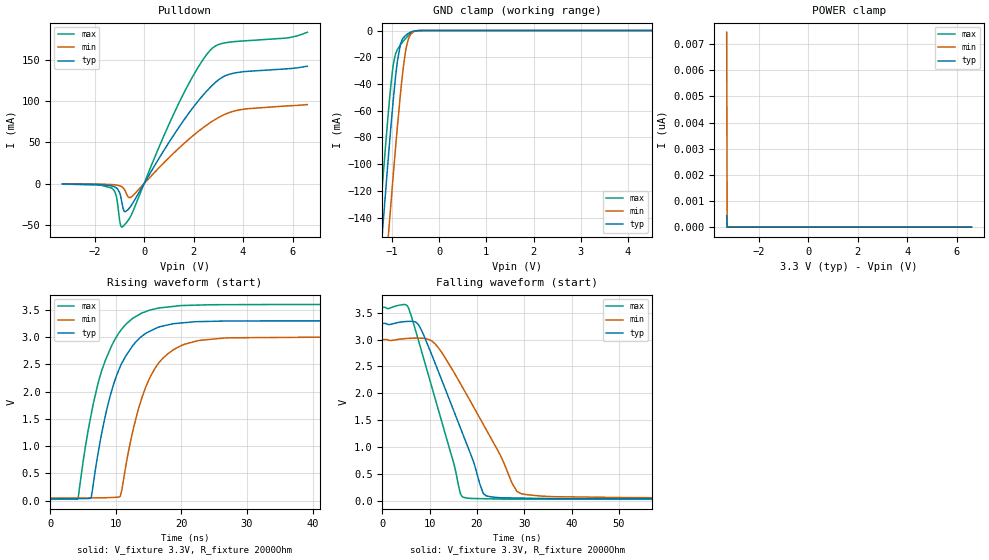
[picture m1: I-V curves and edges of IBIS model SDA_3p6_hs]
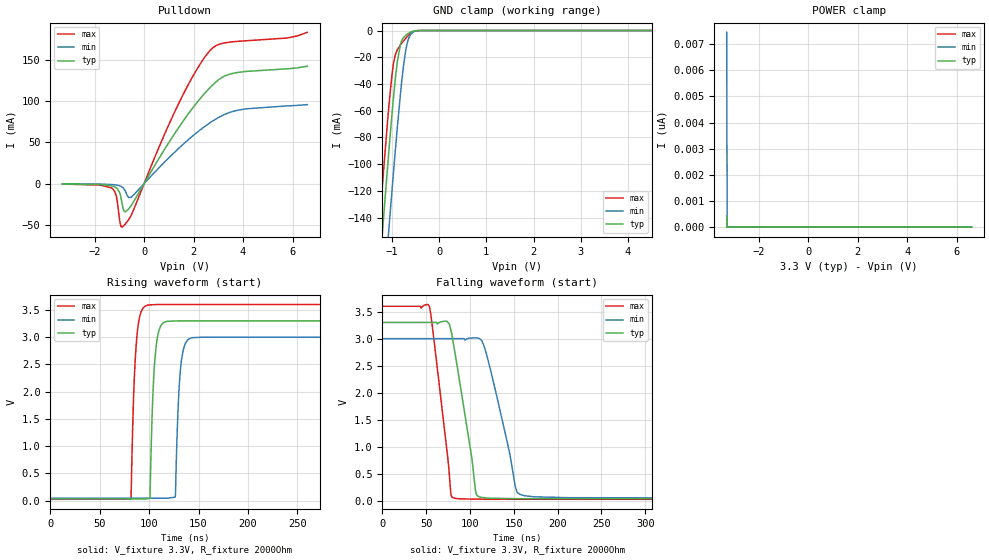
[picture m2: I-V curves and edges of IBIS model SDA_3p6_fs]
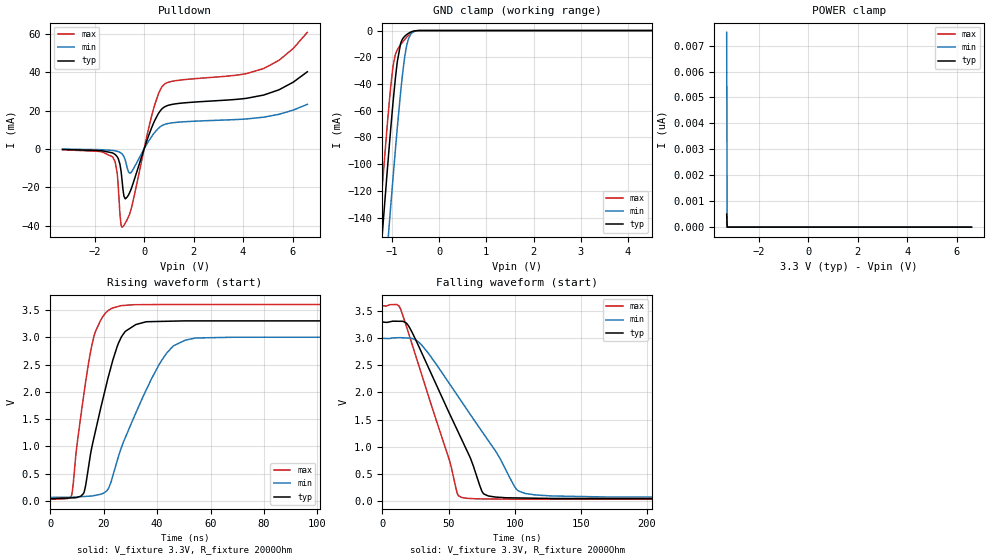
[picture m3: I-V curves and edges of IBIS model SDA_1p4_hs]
|Texas Instruments Incorporated
| Digital Temperature Sensor with Two-Wire Interface and Alert
| Marketing part#   Digital Voltage Range
| TMP75C   1.4V - 3.6V
[IBIS Ver]   4.1
[File name]   tmp75c.ibs
[File Rev]   1.0
[Date]   03/07/2014
[Source]
| Texas Instruments Incorporated.
| 12500 TI Blvd
| Dallas, TX -75243
[Notes]   Revision History:
| Rev 1.1: 09/17/2018
| - SDA_3p6_hs and SDA_3p6_fs models updated.
| Rev 1.0: 03/07/2014
| - Initial version of the model
| - Model generated from simulations in TISPICE
| - C_comp although listed in numerical order of value are
|   obtained from varying PVT conditions. For PVT conditions for
|   each specific value refer the buffer description under
|   respective [Model]. IBIS model user is responsible for using
|   appropriate C_comp to simulate for Signal Integrity.
| - Warnings regarding combined Non-monotonicity of various models have been
|   reviewd and considered minor and can be ignored.
| - Model names with a trailing _1p4 contains the model for
|   1.4V operation.Model names with a trailing _3p6 contains the model
|   for 3.6V operation.
[Disclaimer]
| This model is designed as an aid for customers of Texas Instruments.
| TI and its licensors and suppliers make no warranties, either expressed
| or implied, with respect to this  model, including the warranties of
| merchantability or fitness for a particular purpose. The model is
| provided solely on an "as is" basis. The entire risk as to its quality
| and performance is with the customer.
[Copyright]
 (C) Copyright 2014 Texas Instruments Incorporated.All rights reserved.
|   Device
[Component]   TMP75C
[Manufacturer]   TI
[Package]
| variable   typ   min   max
R_pkg   0.083   0.076   0.088
L_pkg   1.774nH   1.670nH   1.869nH
C_pkg   0.393pF   0.385pF   0.402pF
[Pin]  signal_name   model_name   R_pin   L_pin   C_pin
1   SDA   SDA   0.08836   1.8688nH   0.38537pF
2   SCL   SCL   0.0798   1.72452nH   0.40219pF
3   ALERT   ALERT   0.07626   1.67019nH   0.40077pF
4   GND   GND   0.08804   1.86388nH   0.38801pF
5   A2   A1   0.08833   1.8612nH   0.38619pF
6   A1   A1   0.07742   1.67952nH   0.40007pF
7   A0   A0   0.07743   1.67952nH   0.40011pF
8   V+   POWER   0.08723   1.84409nH   0.38521pF
|   Model Selectors
[Model Selector]  SDA
SDA_3p6_fs   SDA buffer at 3.6V with fast mode.
SDA_3p6_hs   SDA buffer at 3.6V with high speed mode.
SDA_1p4_fs   SDA buffer at 1.4V with fast mode.
SDA_1p4_hs   SDA buffer at 1.4V with high speed mode.
[Model Selector]  SCL
SCL_3p6   SCL buffer at 3.6V.
SCL_1p4   SCL buffer at 1.4V.
[Model Selector]  ALERT
ALERT_3p6   SCL buffer at 3.6V.
ALERT_1p4   SCL buffer at 1.4V.
[Model Selector]  A1
A1_3p6   A1/A2 buffer at 3.6V.
A1_1p4   A1/A2 buffer at 1.4V.
[Model Selector]  A0
A0_3p6   A0 buffer at 3.6V.
A0_1p4   A0 buffer at 1.4V.
| Models and submodels in the file (12): SDA_3p6_hs (I/O_open_drain), SDA_3p6_fs (I/O_open_drain), SDA_1p4_hs (I/O_open_drain), SDA_1p4_fs (I/O_open_drain), SCL_3p6 (Input), SCL_1p4 (Input), ALERT_3p6 (Open_drain), ALERT_1p4 (Open_drain), A1_3p6 (Input), A1_1p4 (Input), A0_3p6 (Input), A0_1p4 (Input)
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|   Model
[Model]   SDA_3p6_hs
Model_type   I/O_open_drain
Polarity   Non-Inverting
Enable   Active-Low
Vinl = 0.5
Vinh = 1.4
Vmeas = 1.65
Vref = 3.3
Cref = 1pF
Rref = 2000
|   typ   min   max
C_comp   0.767pF   0.704pF   0.863pF
[Voltage Range]   3.3   3   3.6
[Temperature Range]   25   125   -40
[Pullup Reference]   3.3   3   3.6
[Pulldown Reference]   0   0   0
[Power Clamp Reference]   3.3   3   3.6
[GND Clamp Reference]   0   0   0
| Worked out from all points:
|   slope of the pulldown table from 0 to 0.495 V, typ, clamps not added: 19.6 ohm
|   GND clamp passes 1 mA (typ) near -0.59 V on its own axis
|   falling waveform, V_fixture 3.3V, R_fixture 2000Ohm: 20-80 % time 8.64ns typ, 11ns min, 7ns max; typ from 3.3 V to 0.031 V
|   rising waveform, V_fixture 3.3V, R_fixture 2000Ohm: 20-80 % time 4.43ns typ, 4.36ns min, 4.49ns max; typ from 0.032 V to 3.3 V
[Pulldown]
|   Voltage   I(typ)   I(min)   I(max)
-3.3V     -437.4uA   -247.2uA   -600.7uA
-1.3V     -2.881mA   -1.227mA   -5.604mA
-1.122V   -5.223mA   -1.809mA   -15.61mA
-973.5mV  -12.58mA   -2.879mA   -47.55mA
-894.3mV  -23.64mA   -4.05mA    -52.74mA
-765.6mV  -34.14mA   -8.745mA   -49.02mA
-518.1mV  -26.42mA   -16.28mA   -38.03mA
1.304V    63.54mA    39.9mA     90.99mA
2.095V    96.47mA    60.83mA    136.3mA
2.68V     116.6mA    73.83mA    161.5mA
3.62V     133.5mA    87.51mA    171.6mA
6.6V      141.9mA    95.47mA    182.9mA
[GND Clamp]
|   Voltage   I(typ)   I(min)   I(max)
-3.3V     -1.174A    -1.231A    -1.141A
-1.29V    -193.5mA   -253.4mA   -157.8mA
-1.251V   -175.1mA   -235mA     -139.4mA
-1.191V   -147.7mA   -207.5mA   -112.3mA
-1.063V   -90.37mA   -149.1mA   -57.03mA
-963.6mV  -49.9mA    -105.8mA   -24.49mA
-884.4mV  -23.47mA   -73.04mA   -14.42mA
-815.1mV  -9.936mA   -46.83mA   -10.7mA
-755.7mV  -5.477mA   -27.58mA   -7.962mA
-696.3mV  -3.35mA    -13.32mA   -5.458mA
-587.4mV  -990.5uA   -2.271mA   -1.777mA
6.6V      0A         0A         0A
[POWER Clamp]
|   Voltage   I(typ)   I(min)   I(max)
-3.3V     435.8pA    7.448nA    127.3pA
-3.28V    0A         0A         0A
-3.27V    0A         0A         0A
6.6V      0A         0A         0A
[Ramp]
R_load = 2000
|   typ   min   max
dV/dt_r   1.96106/4.42647e-09   1.77266/4.35501e-09   2.14571/4.48923e-09
dV/dt_f   1.96115/8.64404e-09   1.77274/1.09923e-08   2.14582/6.99294e-09
[Falling Waveform]
V_fixture = 3.3V
V_fixture_min = 3V
V_fixture_max = 3.6V
R_fixture = 2000Ohm
C_fixture = 0F
|   Time   V(typ)   V(min)   V(max)
0s        3.3V       3V         3.6V
5.492ns   3.338V     3.022V     3.594V
8.291ns   3.169V     3.025V     2.781V
11.4ns    2.502V     2.894V     1.825V
16.49ns   1.357V     2.18V      127.8mV
18.36ns   933.5mV    1.891V     43.02mV
21.91ns   89.91mV    1.329V     34.49mV
28.47ns   47.98mV    170.5mV    27.75mV
33.77ns   40.28mV    82.22mV    26.91mV
500ns     31.41mV    45.42mV    23.64mV
[Rising Waveform]
V_fixture = 3.3V
V_fixture_min = 3V
V_fixture_max = 3.6V
R_fixture = 2000Ohm
C_fixture = 0F
|   Time   V(typ)   V(min)   V(max)
0s        31.57mV    45.57mV    23.82mV
4.194ns   35.33mV    49.26mV    31.49mV
6.247ns   60.07mV    51.06mV    1.588V
8.291ns   1.502V     52.86mV    2.537V
10.66ns   2.46V      78.47mV    3.111V
12.68ns   2.861V     1.328V     3.355V
14.55ns   3.07V      2.085V     3.47V
16.62ns   3.188V     2.54V      3.537V
19.84ns   3.259V     2.838V     3.58V
500ns     3.3V       3V         3.6V
|   Model
[Model]   SDA_3p6_fs
Model_type   I/O_open_drain
Polarity   Non-Inverting
Enable   Active-Low
Vinl = 0.5
Vinh = 1.4
Vmeas = 1.65
Vref = 3.3
Cref = 1pF
Rref = 2000
|   typ   min   max
C_comp   0.767pF   0.704pF   0.863pF
[Voltage Range]   3.3   3   3.6
[Temperature Range]   25   125   -40
[Pullup Reference]   3.3   3   3.6
[Pulldown Reference]   0   0   0
[Power Clamp Reference]   3.3   3   3.6
[GND Clamp Reference]   0   0   0
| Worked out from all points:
|   slope of the pulldown table from 0 to 0.495 V, typ, clamps not added: 19.6 ohm
|   GND clamp passes 1 mA (typ) near -0.59 V on its own axis
|   falling waveform, V_fixture 3.3V, R_fixture 2000Ohm: 20-80 % time 19.1ns typ, 24.2ns min, 15.4ns max; typ from 3.3 V to 0.031 V
|   rising waveform, V_fixture 3.3V, R_fixture 2000Ohm: 20-80 % time 4.44ns typ, 4.36ns min, 4.51ns max; typ from 0.032 V to 3.3 V
[Pulldown]
|   Voltage   I(typ)   I(min)   I(max)
-3.3V     -437.5uA   -247.2uA   -600.7uA
-1.3V     -2.881mA   -1.227mA   -5.604mA
-1.122V   -5.223mA   -1.809mA   -15.61mA
-973.5mV  -12.58mA   -2.879mA   -47.55mA
-894.3mV  -23.64mA   -4.05mA    -52.74mA
-765.6mV  -34.14mA   -8.745mA   -49.02mA
-518.1mV  -26.42mA   -16.28mA   -38.03mA
1.304V    63.54mA    39.9mA     90.99mA
2.095V    96.47mA    60.83mA    136.3mA
2.68V     116.6mA    73.83mA    161.5mA
3.62V     133.5mA    87.51mA    171.6mA
6.6V      141.9mA    95.47mA    182.9mA
[GND Clamp]
|   Voltage   I(typ)   I(min)   I(max)
-3.3V     -1.174A    -1.231A    -1.141A
-1.29V    -193.5mA   -253.4mA   -157.8mA
-1.251V   -175.1mA   -235mA     -139.4mA
-1.191V   -147.7mA   -207.5mA   -112.3mA
-1.063V   -90.37mA   -149.1mA   -57.03mA
-963.6mV  -49.9mA    -105.8mA   -24.49mA
-884.4mV  -23.47mA   -73.04mA   -14.42mA
-815.1mV  -9.936mA   -46.83mA   -10.7mA
-755.7mV  -5.477mA   -27.58mA   -7.962mA
-696.3mV  -3.35mA    -13.32mA   -5.458mA
-587.4mV  -990.5uA   -2.271mA   -1.777mA
6.6V      0A         0A         0A
[POWER Clamp]
|   Voltage   I(typ)   I(min)   I(max)
-3.3V     435.8pA    7.448nA    127.3pA
-3.28V    0A         0A         0A
-3.27V    0A         0A         0A
6.6V      0A         0A         0A
[Ramp]
R_load = 2000
|   typ   min   max
dV/dt_r   1.96106/4.42663e-09   1.77265/4.35276e-09   2.14571/4.4895e-09
dV/dt_f   1.96114/1.90943e-08   1.77254/2.42331e-08   2.14581/1.54182e-08
[Falling Waveform]
V_fixture = 3.3V
V_fixture_min = 3V
V_fixture_max = 3.6V
R_fixture = 2000Ohm
C_fixture = 0F
|   Time   V(typ)   V(min)   V(max)
0s        3.3V       3V         3.6V
53.78ns   3.3V       3V         3.595V
73.62ns   3.323V     3V         935.9mV
78.19ns   3.153V     3V         125.2mV
81.02ns   2.91V      3V         50.32mV
106.4ns   167.2mV    3.015V     28.13mV
110.1ns   74.26mV    3.007V     27.35mV
119.2ns   48.6mV     2.692V     25.49mV
157.8ns   35.43mV    110.2mV    25.3mV
500ns     31.44mV    45.76mV    23.64mV
[Rising Waveform]
V_fixture = 3.3V
V_fixture_min = 3V
V_fixture_max = 3.6V
R_fixture = 2000Ohm
C_fixture = 0F
|   Time   V(typ)   V(min)   V(max)
0s        31.57mV    45.57mV    23.82mV
81.62ns   29.91mV    44.58mV    27.15mV
87.43ns   29.8mV     44.51mV    2.977V
97.77ns   33.31mV    44.39mV    3.584V
106.7ns   2.757V     44.28mV    3.598V
115.5ns   3.277V     44.17mV    3.6V
126.5ns   3.297V     87.5mV     3.6V
131.8ns   3.3V       2.436V     3.6V
142.4ns   3.3V       2.985V     3.6V
500ns     3.3V       3V         3.6V
|   Model
[Model]   SDA_1p4_hs
Model_type   I/O_open_drain
Polarity   Non-Inverting
Enable   Active-Low
Vinl = 0.5
Vinh = 1.4
Vmeas = 0.7
Vref = 3.3
Cref = 1pF
Rref = 2000
|   typ   min   max
C_comp   0.767pF   0.704pF   0.863pF
[Voltage Range]   3.3   3   3.6
[Temperature Range]   25   125   -40
[Pullup Reference]   3.3   3   3.6
[Pulldown Reference]   0   0   0
[Power Clamp Reference]   3.3   3   3.6
[GND Clamp Reference]   0   0   0
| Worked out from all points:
|   slope of the pulldown table from 0 to 0.495 V, typ, clamps not added: 30.1 ohm
|   GND clamp passes 1 mA (typ) near -0.59 V on its own axis
|   falling waveform, V_fixture 3.3V, R_fixture 2000Ohm: 20-80 % time 36.7ns typ, 47.9ns min, 28.2ns max; typ from 3.3 V to 0.041 V
|   rising waveform, V_fixture 3.3V, R_fixture 2000Ohm: 20-80 % time 9.31ns typ, 15.2ns min, 6.34ns max; typ from 0.041 V to 3.3 V
[Pulldown]
|   Voltage   I(typ)   I(min)   I(max)
-3.3V     -298.9uA   -147.7uA   -425.1uA
-1.27V    -2.144mA   -818.9uA   -4.265mA
-1.092V   -4.054mA   -1.248mA   -12.49mA
-973.5mV  -8.327mA   -1.847mA   -34.77mA
-894.3mV  -16.17mA   -2.614mA   -40.84mA
-815.1mV  -24.75mA   -4.104mA   -39.85mA
-636.9mV  -24.13mA   -11.85mA   -35.55mA
-498.3mV  -19.99mA   -11.83mA   -30.05mA
323.4mV   11.68mA    6.808mA    18.15mA
768.9mV   21.42mA    12.48mA    33.13mA
4.838V    28.11mA    16.55mA    41.95mA
6.6V      40.24mA    23.26mA    60.83mA
[GND Clamp]
|   Voltage   I(typ)   I(min)   I(max)
-3.3V     -1.174A    -1.231A    -1.141A
-1.29V    -193.5mA   -253.4mA   -157.8mA
-1.251V   -175.1mA   -235mA     -139.4mA
-1.191V   -147.7mA   -207.5mA   -112.3mA
-1.063V   -90.37mA   -149.1mA   -57.03mA
-963.6mV  -49.9mA    -105.8mA   -24.49mA
-884.4mV  -23.47mA   -73.04mA   -14.42mA
-815.1mV  -9.937mA   -46.83mA   -10.7mA
-755.7mV  -5.477mA   -27.58mA   -7.962mA
-696.3mV  -3.35mA    -13.32mA   -5.458mA
-587.4mV  -990.5uA   -2.271mA   -1.777mA
6.6V      0A         0A         0A
[POWER Clamp]
|   Voltage   I(typ)   I(min)   I(max)
-3.3V     501.8pA    7.511nA    196.3pA
-3.28V    0A         0A         0A
-3.27V    0A         0A         0A
6.6V      0A         0A         0A
[Ramp]
R_load = 2000
|   typ   min   max
dV/dt_r   1.95536/9.28248e-09   1.76173/1.52025e-08   2.14269/6.30924e-09
dV/dt_f   1.95536/3.67127e-08   1.76171/4.79306e-08   2.14269/2.82704e-08
[Falling Waveform]
V_fixture = 3.3V
V_fixture_min = 3V
V_fixture_max = 3.6V
R_fixture = 2000Ohm
C_fixture = 0F
|   Time   V(typ)   V(min)   V(max)
0s        3.3V       3V         3.6V
13.72ns   3.313V     3.011V     3.543V
20.15ns   3.215V     3.004V     3.067V
29.74ns   2.731V     2.874V     2.327V
56.55ns   1.309V     1.951V     142.1mV
59.89ns   1.135V     1.831V     64.22mV
76.85ns   125.9mV    1.225V     37.01mV
100.5ns   55.15mV    240.4mV    30.87mV
108.2ns   52.26mV    136.2mV    30.83mV
500ns     41.06mV    63.81mV    28.85mV
[Rising Waveform]
V_fixture = 3.3V
V_fixture_min = 3V
V_fixture_max = 3.6V
R_fixture = 2000Ohm
C_fixture = 0F
|   Time   V(typ)   V(min)   V(max)
0s        41.06mV    63.78mV    28.85mV
7.97ns    55.13mV    67.62mV    103.2mV
12.52ns   143.7mV    80.4mV     1.935V
17.02ns   1.303V     103.2mV    3.12V
21.64ns   2.258V     217.5mV    3.487V
26.56ns   3V         968.3mV    3.579V
32.02ns   3.233V     1.612V     3.596V
43.54ns   3.292V     2.708V     3.6V
54.49ns   3.3V       2.986V     3.6V
500ns     3.3V       3V         3.6V
